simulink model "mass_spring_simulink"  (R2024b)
settings: Solver=VariableStepAuto  StartTime=0.0  StopTime=20  MaxStep=0.01  RelTol=1e-3

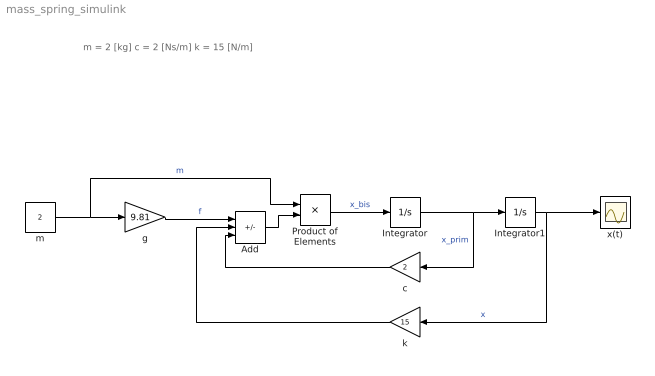
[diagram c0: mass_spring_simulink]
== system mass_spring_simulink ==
  note: m = 2 [kg] c = 2 [Ns/m] k = 15 [N/m]
  Add : Sum  Inputs=+--
  Integrator : Integrator
  Integrator1 : Integrator
  Product of Elements : Product  Inputs=/*
  c : Gain  Gain=2
  g : Gain  Gain=9.81
  k : Gain  Gain=15
  m : Constant  Value=2
  x(t) : Scope
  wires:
  Integrator/1 -> c/1, Integrator1/1  "x_prim"
  Product of Elements/1 -> Integrator/1  "x_bis"
  Integrator1/1 -> k/1, x(t)/1  "x"
  m/1 -> Product of Elements/1, g/1  "m"
  c/1 -> Add/3
  k/1 -> Add/2
  g/1 -> Add/1  "f"
  Add/1 -> Product of Elements/2
